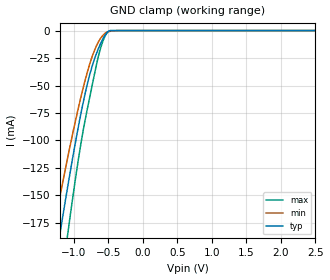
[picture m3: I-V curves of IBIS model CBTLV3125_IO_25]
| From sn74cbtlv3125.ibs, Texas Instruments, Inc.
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[Model]   CBTLV3125_IO_25
Model_type  Terminator
| variable   typ   min   max
C_comp   5.30pF   4.50pF   5.91pF
| C_tri-state   5.30pF   4.50pF   5.91pF
[Temperature Range]   40   100   -40
| Ambient temperature   25   85   -40
[Voltage range]   2.5   2.3   2.7
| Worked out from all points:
|   GND clamp passes 1 mA (typ) near -0.51 V on its own axis
[GND Clamp]
| CBTLV3125_IO_25
|   Voltage   I(typ)   I(min)   I(max)
-2.5V     -744.7mA   -617.6mA   -935mA
-1.295V   -221.3mA   -181.1mA   -284.7mA
-1.205V   -185.7mA   -151.6mA   -240.1mA
-1.175V   -174.1mA   -141.9mA   -225.5mA
-1.085V   -140mA     -113.8mA   -182.7mA
-915mV    -80.62mA   -64.72mA   -108.9mA
-795mV    -45.89mA   -35.43mA   -67.85mA
-715mV    -28.24mA   -20.04mA   -43.47mA
-640mV    -15.52mA   -9.679mA   -22.02mA
-535mV    -2.819mA   -1.87mA    -3.407mA
-475mV    -81.98uA   -648uA     -50.52uA
2.5V      1.258nA    61.07nA    12.6pA
